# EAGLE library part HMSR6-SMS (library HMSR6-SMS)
Current Sensor 6A 1 Channel Hall Effect, Open Loop Bidirectional 16-PowerSOIC (0.295", 7.50mm Width), 10 Leads Source: Datasheet
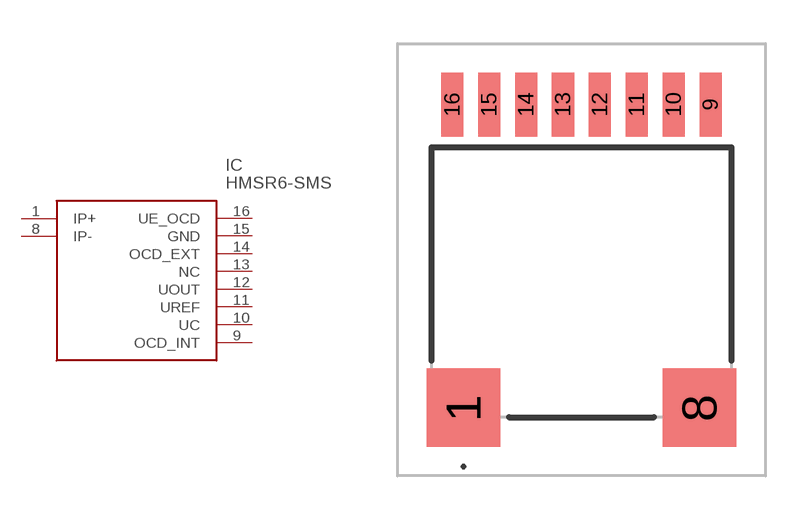
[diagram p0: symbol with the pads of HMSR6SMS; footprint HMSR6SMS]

Designator prefix IC

## HMSR6-SMS (Description: Current Sensor 6A 1 Channel Hall Effect, Open Loop Bidirectional 16-PowerSOIC (0.295", 7.50mm Width), 10 Leads; Height: 6.25mm; Manufacturer_Name: LEM; Manufacturer_Part_Number: HMSR6-SMS)  [HMSR6SMS]
1  IP+
8  IP-
9  OCD_INT
10  UC
11  UREF
12  UOUT
13  NC  nc
14  OCD_EXT
15  GND
16  UE_OCD

## Footprint HMSR6SMS (pad centres in mm)
10.32x9.3x6.1mm
smd 2.54 x 2.7: 1 -4.06,-4.325; 8 4.06,-4.325
smd 0.76 x 2.2: 9 4.445,6.125; 10 3.175,6.125; 11 1.905,6.125; 12 0.635,6.125; 13 -0.635,6.125; 14 -1.905,6.125; 15 -3.175,6.125; 16 -4.445,6.125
